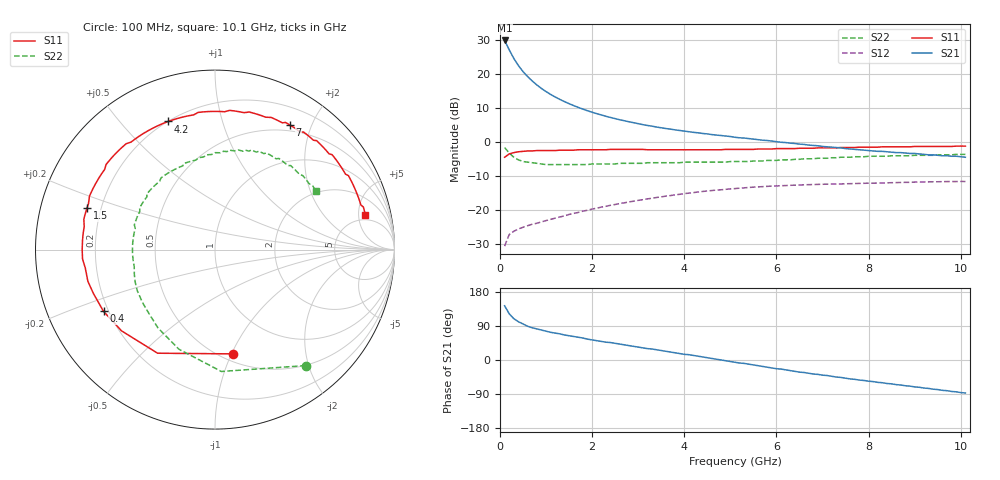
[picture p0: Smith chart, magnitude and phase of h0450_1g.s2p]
!HBFP-0450
!S and NOISE PARAMETERS at Vce=1V  Ic=35mA.  LAST UPDATED  09-04-98
# GHZ S MA R  50
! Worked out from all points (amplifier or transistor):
!   101 points, 100 MHz to 10.1 GHz, reference 50 ohm
!   highest |S21| = 29.8 dB at 100 MHz (marker M1)
!   |S21| within 3 dB of that: start of sweep to 209.8 MHz
!   unconditionally stable (mu >= 1): 2.155 GHz to end of sweep
!   at 1.7 GHz: K = 0.93, MSG = 15.4 dB, |S12| = -20.8 dB
!   at 5.1 GHz: K = 1.10, MAG = 5.6 dB, |S12| = -13.8 dB
!   at 10.1 GHz: K = 1.09, MAG = 1.8 dB, |S12| = -11.7 dB
!   lowest NFmin = 1.50 dB at 1.8 GHz
!   S11 on the Smith chart (normalised r, x): 100 MHz: 0.57, -1.02; 400 MHz: 0.18, -0.25; 1.5 GHz: 0.15, +0.16; 4.2 GHz: 0.20, +0.68; 7 GHz: 0.42, +1.69; 10.1 GHz: 4.09, +6.08
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0.1  0.59 -80.0  30.83 143.0  0.029 59.0  0.82 -52.0
0.2  0.66 -119.0  22.46 122.0  0.043 44.0  0.68 -87.0
0.3  0.69 -139.0  16.75 109.0  0.048 37.0  0.59 -110.0
0.4  0.71 -151.0  13.15 101.0  0.052 34.0  0.54 -126.0
0.5  0.72 -160.0  10.73 95.0  0.055 32.0  0.51 -137.0
0.6  0.73 -166.0  9.07 89.0  0.058 31.0  0.5 -144.0
0.7  0.73 -172.0  7.8 85.0  0.061 32.0  0.49 -152.0
0.8  0.74 -176.0  6.83 82.0  0.063 32.0  0.48 -158.0
0.9  0.74 180.0  6.06 79.0  0.066 33.0  0.47 -163.0
1.1  0.74 173.0  4.95 73.0  0.072 34.0  0.46 -172.0
1.3  0.75 167.0  4.18 69.0  0.078 34.0  0.46 -179.0
1.5  0.75 162.0  3.62 64.0  0.085 34.0  0.46 175.0
1.8  0.76 155.0  3.01 58.0  0.095 34.0  0.46 167.0
2.3  0.76 144.0  2.36 47.0  0.112 31.0  0.47 157.0
3  0.77 131.0  1.84 34.0  0.137 25.0  0.48 144.0
3.5  0.76 122.0  1.6 25.0  0.154 20.0  0.49 136.0
4.2  0.76 110.0  1.37 12.0  0.178 11.0  0.5 124.0
5.1  0.77 93.0  1.16 -6.0  0.204 -2.0  0.51 108.0
6.8  0.8 62.0  0.88 -37.0  0.234 -27.0  0.56 79.0
7  0.81 59.0  0.85 -40.0  0.236 -29.0  0.57 76.0
8.5  0.84 36.0  0.7 -63.0  0.249 -49.0  0.62 55.0
10.1  0.86 13.0  0.59 -87.0  0.259 -72.0  0.65 30.0
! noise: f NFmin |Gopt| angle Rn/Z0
1.8  1.5  0.59  -155  0.07
2  1.55  0.6  -152  0.08
2.5  1.66  0.61  -143  0.13
3.5  1.94  0.65  -125  0.27
4  2.11  0.67  -115  0.41
5  2.33  0.7  -95  0.75
5.5  2.49  0.72  -85  1.04
7  2.85  0.75  -57  2.09
8  3.14  0.79  -41  2.95
10  3.63  0.81  -12  4.49
